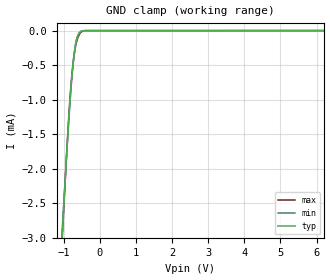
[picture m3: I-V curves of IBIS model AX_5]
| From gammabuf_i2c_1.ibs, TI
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|   Input AX model 5V
[Model]   AX_5
Model_type   Input
|Signals   A0, A1, LD
Vinl = 1.5
Vinh = 3.5
|   typ   min   max
C_comp   6.1203700e-12   7.3057800e-12  5.0777520e-12
[Voltage Range]   5   4.75   5.25
[Temperature Range]   27   85   -40
[Power Clamp Reference]   5   4.75   5.25
[GND Clamp Reference]   0   0   0
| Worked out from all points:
|   GND clamp passes 1 mA (typ) near -0.82 V on its own axis
[GND Clamp]
|   Voltage   I(typ)   I(min)   I(max)
-5V       -45.96mA   -43.01mA   -50.22mA
-1.089V   -3.411mA   -3.309mA   -3.534mA
-1.032V   -2.851mA   -2.785mA   -2.929mA
-936.2mV  -1.946mA   -1.928mA   -1.939mA
-861.1mV  -1.296mA   -1.304mA   -1.239mA
-814.4mV  -934.5uA   -946.7uA   -877.4uA
-764.8mV  -600.7uA   -617.8uA   -584uA
-715.4mV  -353.2uA   -362.7uA   -369.3uA
-659.5mV  -156.3uA   -173.9uA   -199uA
-608mV    -67.3uA    -74.91uA   -106.5uA
-519.2mV  -9.081uA   -11.8uA    -22.05uA
9.985V    0A         0A         0A
[POWER Clamp]
|   Voltage   I(typ)   I(min)   I(max)
-5V       0A         0A         0A
0V        0A         0A         0A
10V       0A         0A         0A
